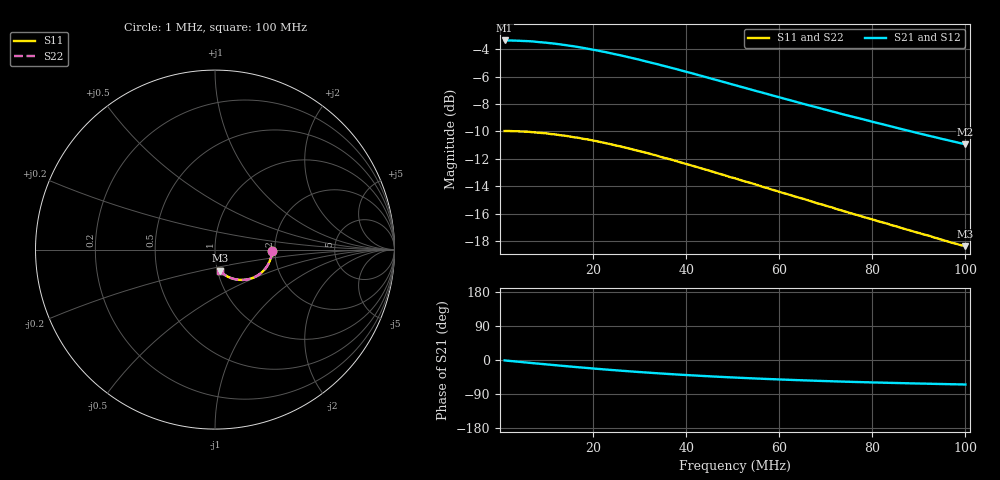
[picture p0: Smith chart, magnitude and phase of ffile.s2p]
# Hz S RI R 50.0
! written by SimSmith version 18.3c
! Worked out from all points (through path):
!   101 points, 1 MHz to 100 MHz, reference 50 ohm
!   highest |S21| = -3.37 dB at 1 MHz (marker M1); lowest = -10.9 dB at 100 MHz (marker M2)
!   group delay of S21, straight-line fit = 1.72 ns
!   lowest |S11| = -18.4 dB at 100 MHz (marker M3), VSWR 1.27, Z = 51.2 - j12.2 ohm
!   |S11| at or under -10 dB: 4.242 MHz to end of sweep
!   |S22| runs from -18.4 to -10.0 dB; largest |S21 - S12| = 0
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1000000  0.3171 -0.00706  0.6783 -0.0137  0.6783 -0.0137  0.3171 -0.00706
2980000  0.3161 -0.0207  0.6765 -0.0412  0.6765 -0.0412  0.3161 -0.0207
5950000  0.3128 -0.0412  0.6696 -0.0817  0.6696 -0.0817  0.3128 -0.0412
8920000  0.3061 -0.0609  0.6571 -0.1203  0.6571 -0.1203  0.3061 -0.0609
1.288e7  0.2942 -0.0854  0.6348 -0.1682  0.6348 -0.1682  0.2942 -0.0854
1.585e7  0.2835 -0.1014  0.6142 -0.2004  0.6142 -0.2004  0.2835 -0.1014
1.783e7  0.2754 -0.1117  0.5987 -0.2196  0.5987 -0.2196  0.2754 -0.1117
2.278e7  0.2539 -0.1326  0.5562 -0.2615  0.5562 -0.2615  0.2539 -0.1326
2.575e7  0.24 -0.1427  0.5295 -0.2815  0.5295 -0.2815  0.24 -0.1427
2.971e7  0.2207 -0.153  0.4932 -0.3027  0.4932 -0.3027  0.2207 -0.153
3.466e7  0.1967 -0.162  0.4477 -0.3211  0.4477 -0.3211  0.1967 -0.162
3.862e7  0.1789 -0.1664  0.4133 -0.3307  0.4133 -0.3307  0.1789 -0.1664
4.159e7  0.1662 -0.1681  0.3889 -0.3351  0.3889 -0.3351  0.1662 -0.1681
4.654e7  0.1457 -0.169  0.3502 -0.3381  0.3502 -0.3381  0.1457 -0.169
5.05e7  0.1314 -0.1681  0.3219 -0.3372  0.3219 -0.3372  0.1314 -0.1681
5.842e7  0.1047 -0.1633  0.2722 -0.3306  0.2722 -0.3306  0.1047 -0.1633
6.733e7  0.0808 -0.1549  0.226 -0.3177  0.226 -0.3177  0.0808 -0.1549
7.624e7  0.0614 -0.1451  0.1889 -0.3019  0.1889 -0.3019  0.0614 -0.1451
8.416e7  0.0472 -0.1359  0.1626 -0.2864  0.1626 -0.2864  0.0472 -0.1359
9.01e7  0.0384 -0.1291  0.1453 -0.2747  0.1453 -0.2747  0.0384 -0.1291
9.703e7  0.0294 -0.1207  0.1282 -0.2618  0.1282 -0.2618  0.0294 -0.1207
1e8  0.0259 -0.1178  0.1215 -0.2566  0.1215 -0.2566  0.0259 -0.1178
